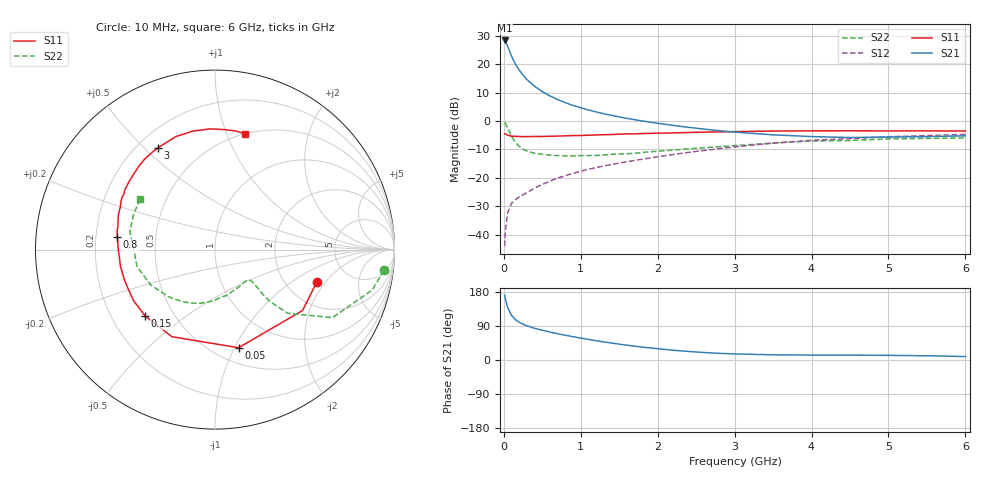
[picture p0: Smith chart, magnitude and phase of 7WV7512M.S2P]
! Infineon Technologies  Discrete & RF Semiconductors
! BFS17W
! Si NPN RF Bipolar Junction Transistor in SOT323
! VCE = 0.75 V  IC = 12 mA
! Common Emitter S-Parameters:  August  1999
# GHz  S  MA  R  50
!  f  S11  S21  S12  S22
! GHz  MAG  ANG  MAG  ANG  MAG  ANG  MAG  ANG
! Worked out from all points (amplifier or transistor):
!   36 points, 10 MHz to 6 GHz, reference 50 ohm
!   highest |S21| = 28.3 dB at 10 MHz (marker M1)
!   |S21| within 3 dB of that: start of sweep to 63.15 MHz
!   unconditionally stable (mu >= 1): 249.1 MHz to end of sweep
!   at 250 MHz: K = 1.00, MAG = 20.7 dB, |S12| = -26.0 dB
!   at 1.4 GHz: K = 1.41, MAG = 4.9 dB, |S12| = -15.3 dB
!   at 6 GHz: K = 1.13, MAG = -2.5 dB, |S12| = -4.7 dB
!   S11 on the Smith chart (normalised r, x): 10 MHz: 2.93, -1.64; 50 MHz: 0.65, -1.04; 150 MHz: 0.34, -0.36; 800 MHz: 0.29, +0.06; 3 GHz: 0.28, +0.55; 6 GHz: 0.50, +1.16
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0.01  0.5952 -17.7  26.1 170.8  0.0063 82.0  0.9484 -7.0
0.02  0.5942 -34.9  25.21 161.0  0.0116 75.4  0.9046 -14.4
0.05  0.5622 -76.5  20.48 138.6  0.0246 60.5  0.7562 -30.1
0.1  0.5414 -116.3  13.85 117.8  0.0357 49.0  0.5383 -41.2
0.15  0.537 -136.6  10.07 106.5  0.0413 47.3  0.4208 -43.4
0.2  0.5355 -148.1  7.838 99.5  0.0462 48.6  0.3589 -43.0
0.25  0.5309 -156.1  6.378 94.4  0.0504 49.9  0.3192 -41.9
0.3  0.532 -161.8  5.368 90.3  0.055 52.5  0.2975 -41.3
0.4  0.535 -170.2  4.078 83.7  0.0662 55.4  0.2694 -40.8
0.5  0.5346 -175.6  3.292 78.5  0.0769 57.5  0.2588 -41.1
0.6  0.5395 179.9  2.751 73.7  0.0876 59.1  0.2507 -42.6
0.7  0.5429 176.1  2.382 69.3  0.0993 60.0  0.2467 -45.3
0.8  0.5491 172.5  2.101 65.3  0.1093 60.6  0.2438 -48.5
1.1  0.5632 163.6  1.564 54.2  0.142 61.0  0.2473 -59.4
1.3  0.5751 158.0  1.342 47.6  0.1625 60.6  0.2518 -68.0
1.6  0.5937 150.9  1.114 39.1  0.1926 59.9  0.2655 -80.6
2.2  0.618 137.1  0.838 25.8  0.2577 57.6  0.3096 -105.1
3  0.6505 119.2  0.639 16.0  0.351 51.4  0.3689 -134.5
3.5  0.6663 109.2  0.571 13.7  0.409 46.0  0.4092 -151.4
4.5  0.6732 92.3  0.512 12.9  0.4907 33.6  0.4542 178.4
5.5  0.6709 80.3  0.532 11.2  0.5549 23.1  0.4949 156.1
6  0.6677 75.6  0.549 9.1  0.582 18.0  0.5028 146.1
